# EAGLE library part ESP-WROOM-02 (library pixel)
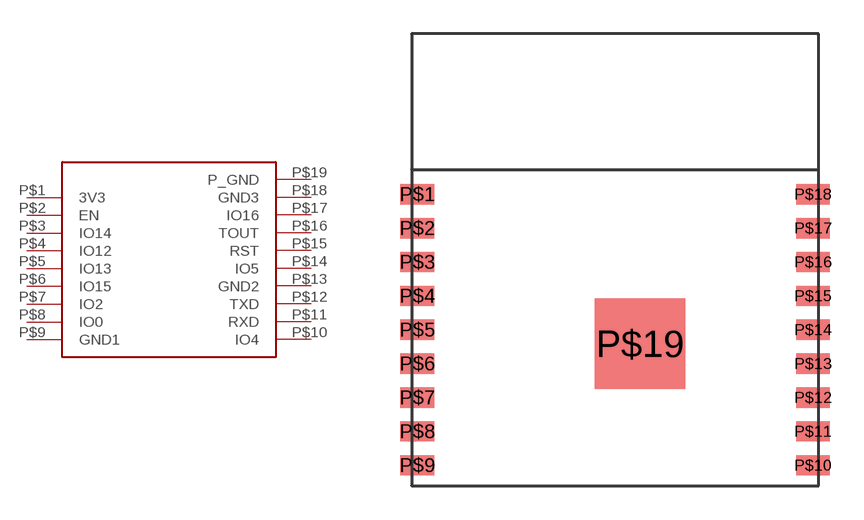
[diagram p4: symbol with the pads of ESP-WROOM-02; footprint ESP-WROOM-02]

Designator prefix -

## ESP-WROOM-02  [ESP-WROOM-02]
P$1  3V3
P$2  EN
P$3  IO14
P$4  IO12
P$5  IO13
P$6  IO15
P$7  IO2
P$8  IO0
P$9  GND1
P$10  IO4
P$11  RXD
P$12  TXD
P$13  GND2
P$14  IO5
P$15  RST
P$16  TOUT
P$17  IO16
P$18  GND3
P$19  P_GND

## Footprint ESP-WROOM-02 (pad centres in mm)
smd 1.5 x 0.9: P$1 -8.75,0; P$2 -8.75,-1.5; P$3 -8.75,-3; P$4 -8.75,-4.5; P$5 -8.75,-6; P$6 -8.75,-7.5; P$7 -8.75,-9; P$8 -8.75,-10.5; P$9 -8.75,-12; P$10 8.75,-12; P$11 8.75,-10.5; P$12 8.75,-9; P$13 8.75,-7.5; P$14 8.75,-6; P$15 8.75,-4.5; P$16 8.75,-3; P$17 8.75,-1.5; P$18 8.75,0
smd 4 x 4: P$19 1.1,-6.61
